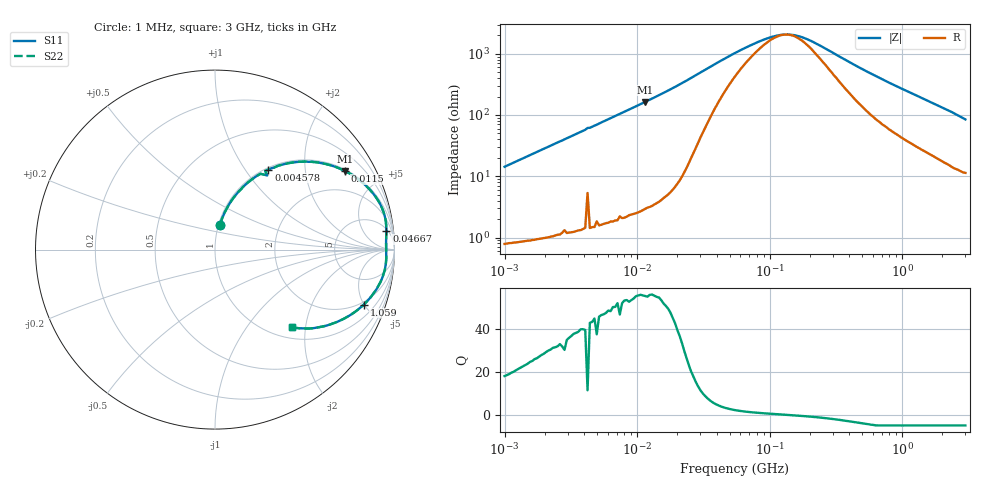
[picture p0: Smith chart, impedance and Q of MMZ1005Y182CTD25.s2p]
! S-Parameter Data Generated by TDK Corporation
! Copyright(C) 2025 TDK Corporation.
! All Rights Reserved.
! TDK P/N: MMZ1005Y182CTD25 (Chip Bead)
! Property: |Z|=1800ohm at 100MHz
! Size(LxWxT): 1x0.5x0.5mm
! Model Type: s2p (Touchstone File Format Version 1.0)
! Frequency: DC=Yes Start=1MHz Stop=3000MHz 202points Log-sweep
! Model Generated on Feb. 6, 2025
! Terms and conditions regarding TDK Simulation Models:
! 1)This simulation model is being provided solely for informational
!  purposes. Please refer to the specifications of the products in
!  terms of detailed characteristics of such products.
! 2)In no event shall TDK Corporation of any of its subsidiaries be
!  liable for any loss or damage arising, directly or indirectly,
!  from any information contained in this simulation model, including,
!  but not limited to loss or damages arising from any inaccuracies,
!  omissions or errors in connection with such information.
! 3)Any and all copyrights on this simulation model are owned by
!  TDK Corporation.  Duplication or redistribution of this simulation
!  model without prior written permission from TDK Corporation
!  is prohibited.
! 4)This simulation model is subject to any modification or change
!  without any prior notice.
! 5)Neither TDK Corporation nor any of its subsidiaries shall make any
!  warranty, express or implied, including but not limited to the
!  correctness, implied warranties of merchantability and fitness for
!  a particular purpose with respect to this simulation models.
! 6)The use of this simulation model shall be deemed to have consented
!  to the terms and conditions hereof.
! Port Assignments:
!  1 ---@@@--- 2
! Applicable Conditions:
!  Temperature = 25 degC
!  DC Bias Current = 0 A
!  Small Signal Operation
# Hz S MA R 50
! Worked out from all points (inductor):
!   201 points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, 1 MHz to 3 GHz, reference 50 ohm
!   read as one part in series: L = 2.27 uH near 1.041 MHz
!   highest Q = 56 at 11.5 MHz (marker M1), where L = 2.26 uH
!   self-resonance near 132.4 MHz
!   S11 on the Smith chart (normalised r, x): 1 MHz: 1.02, +0.29; 4.578 MHz: 1.03, +1.29; 11.5 MHz: 1.06, +3.27; 46.67 MHz: 6, +16; 1.059 GHz: 1.78, -4.98; 3 GHz: 1.23, -1.68
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1000000  0.1405 78.8  0.9824 -8.1  0.9824 -8.1  0.1405 78.8
2139570  0.2882 71.4  0.948 -16.7  0.948 -16.7  0.2882 71.4
2947212  0.3807 66.0  0.9139 -22.4  0.9139 -22.4  0.3807 66.0
3900413  0.4784 60.0  0.8663 -28.6  0.8663 -28.6  0.4784 60.0
4225536  0.505 54.8  0.8204 -30.2  0.8204 -30.2  0.505 54.8
4577760  0.536 56.3  0.832 -32.4  0.832 -32.4  0.536 56.3
7110411  0.701 44.4  0.6999 -44.5  0.6999 -44.5  0.701 44.4
1.149534e7  0.8462 31.2  0.5179 -57.8  0.5179 -57.8  0.8462 31.2
1.461624e7  0.897 25.2  0.426 -63.7  0.426 -63.7  0.897 25.2
2.459509e7  0.9577 14.4  0.2495 -73.1  0.2495 -73.1  0.9577 14.4
4.666789e7  0.9602 6.2  0.1128 -66.3  0.1128 -66.3  0.9602 6.2
5.477226e7  0.9577 4.9  0.09318 -60.6  0.09318 -60.6  0.9577 4.9
8.507507e7  0.9539 2.2  0.05902 -37.5  0.05902 -37.5  0.9539 2.2
1.219755e8  0.9536 0.4  0.04687 -8.0  0.04687 -8.0  0.9536 0.4
1.550909e8  0.9543 -0.8  0.04758 15.6  0.04758 15.6  0.9543 -0.8
2.136344e8  0.9554 -2.5  0.06154 42.4  0.06154 42.4  0.9554 -2.5
4.570858e8  0.9488 -8.4  0.1522 66.2  0.1522 66.2  0.9488 -8.4
8.005644e8  0.916 -15.6  0.2731 64.5  0.2731 64.5  0.916 -15.6
1.059487e9  0.8837 -20.3  0.351 60.8  0.351 60.8  0.8837 -20.3
1.782824e9  0.7844 -31.2  0.5231 51.0  0.5231 51.0  0.7844 -31.2
2.455801e9  0.6887 -39.6  0.6432 43.1  0.6432 43.1  0.6887 -39.6
3e9  0.6074 -45.3  0.7171 37.0  0.7171 37.0  0.6074 -45.3
